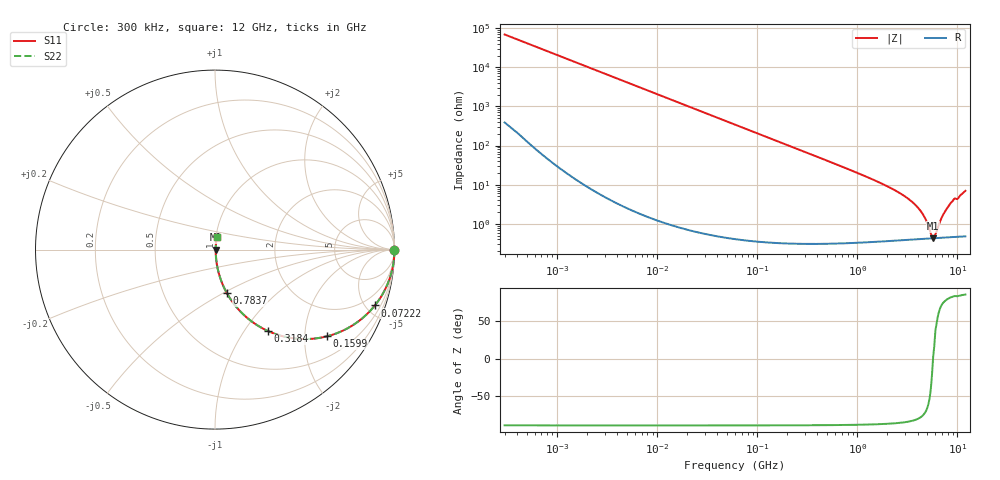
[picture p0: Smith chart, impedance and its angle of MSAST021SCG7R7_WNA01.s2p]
! MSAST021SCG7R7_WNA01  S-PARAMETER MODEL  ( General Type )
! Model Generated by TAIYO YUDEN Corporation (http://www.ty-top.com)
! Version 2.0
! TAIYO YUDEN Control No. 181101
! Copyright(c) 2015 TAIYO YUDEN CO.,LTD. All Rights Reserved.
! Product Description (link to TY-COMPAS)
! https://ds.yuden.co.jp/TYCOMPAS/or/detail?pn=MSAST021SCG7R7CWNA01&u=M
! Products Name : Multilayer Ceramic Capacitors
! Characteristics :
!  Capacitance : 7.7 pF , Rated Voltage : 25V , TCC : CG / C0G
!  Case Size : 0.25 x 0.125 / 0.0098 x 0.0049 [mm/inch] , Thickness : 0.125 / 0.0049 [mm/inch]
!  (Conditions: Temperature = 25 degC , DC Bias Current/Voltage = 0A / 0V)
! External Node Assignments :
!  1  o---| |---o  2
! GND o---------o GND
! Frequency Range : 0.3MHz  -  12000MHz  [ 401 STEP ]
# MHz S RI R 50
! Freq[MHz].  S11 Real  S11 Imag  S21 Real  S21 Imag  S12 Real  S12 Imag  S22 Real  S22 Imag
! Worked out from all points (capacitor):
!   401 points, 300 kHz to 12 GHz, reference 50 ohm
!   read as one part in series: C = 7.7 pF near 316.3 kHz
!   lowest |Z| = 429 mohm at 5.715 GHz (marker M1)
!   series resonance near 5.705 GHz, so ESL is about 100 pH
!   S11 on the Smith chart (normalised r, x): 300 kHz: open; 72.22 MHz: 1.01, -5.72; 159.9 MHz: 1.01, -2.58; 318.4 MHz: 1.01, -1.29; 783.7 MHz: 1.01, -0.52; 12 GHz: 1.01, +0.14
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0.3  1 -0.00145  1.03e-05 0.00145  1.03e-05 0.00145  1 -0.00145
1.769972  0.9999 -0.00856  8.12e-05 0.00856  8.12e-05 0.00856  0.9999 -0.00856
10.44266  0.9974 -0.0504  0.00258 0.0504  0.00258 0.0504  0.9974 -0.0504
27.10171  0.983 -0.1289  0.017 0.1289  0.017 0.1289  0.983 -0.1289
60  0.922 -0.2676  0.078 0.2676  0.078 0.2676  0.922 -0.2676
72.22496  0.8908 -0.3112  0.1092 0.3112  0.1092 0.3112  0.8908 -0.3112
107.4644  0.7867 -0.4088  0.2133 0.4088  0.2133 0.4088  0.7867 -0.4088
159.8975  0.6249 -0.4829  0.3751 0.4829  0.3751 0.4829  0.6249 -0.4829
318.4019  0.2961 -0.4542  0.7039 0.4542  0.7039 0.4542  0.2961 -0.4542
353.9943  0.2539 -0.4326  0.7461 0.4326  0.7461 0.4326  0.2539 -0.4326
783.7017  0.0654 -0.2411  0.9346 0.2411  0.9346 0.2411  0.0654 -0.2411
2088.533  0.0108 -0.0844  0.9892 0.0844  0.9892 0.0844  0.0108 -0.0844
3026.31  0.00622 -0.0486  0.9938 0.0486  0.9938 0.0486  0.00622 -0.0486
3944.255  0.00476 -0.0271  0.9952 0.0271  0.9952 0.0271  0.00476 -0.0271
4623.766  0.00436 -0.0152  0.9956 0.0152  0.9956 0.0152  0.00436 -0.0152
5420.343  0.00425 -0.00362  0.9958 0.00362  0.9958 0.00362  0.00425 -0.00362
5715.274  0.00427 0.000123  0.9957 -0.000123  0.9957 -0.000123  0.00427 0.000123
6026.253  0.00432 0.00335  0.9957 -0.00335  0.9957 -0.00335  0.00432 0.00335
7064.448  0.00464 0.0149  0.9954 -0.0149  0.9954 -0.0149  0.00464 0.0149
8281.503  0.00539 0.0294  0.9946 -0.0294  0.9946 -0.0294  0.00539 0.0294
8966.534  0.00602 0.0379  0.994 -0.0379  0.994 -0.0379  0.00602 0.0379
12000  0.00954 0.0687  0.9905 -0.0687  0.9905 -0.0687  0.00954 0.0687
